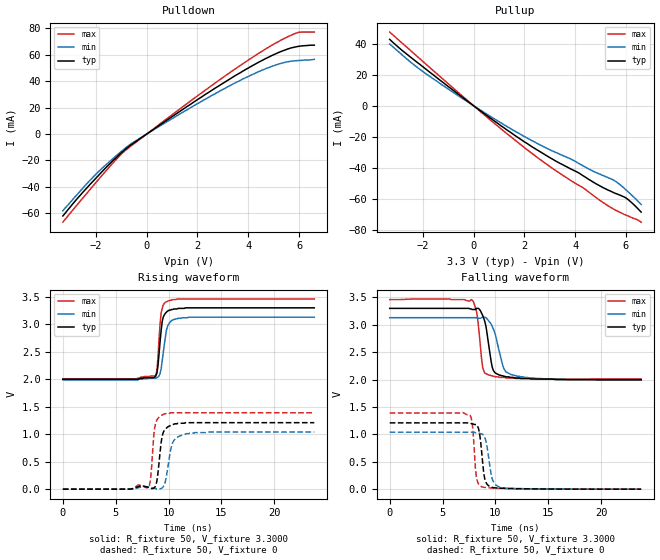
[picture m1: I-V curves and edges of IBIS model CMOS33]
|   IBIS Models For TG-5511CB (CMOS)
[IBIS Ver]   3.2
[File name]   tg5511cb_cmos.ibs
[File Rev]   1.0
[Date]   Feb 10, 2021
[Source]   From silicon level SPICE model at Seiko Epson.
[Notes]
[Disclaimer]
This information is for modeling purposes only, and is not guaranteed.
Property of SEIKO EPSON Corp.,
unauthorized reproduction and/or distribution is strictly prohibited.
[Copyright]   Copyright 2021, SEIKO EPSON Corp. All rights reserved.
[Component]   TG-5511CB (CMOS)
[Manufacturer] SEIKO EPSON Corp.
[Package]
| variable   typ   min   max
R_pkg   0.10   NA   NA
L_pkg   1.47n   NA   NA
C_pkg   0.81p   NA   NA
[Pin] signal_name   model_name   R_pin  L_pin  C_pin
  4   GND   GND   NA   NA   NA
  5   OUT   CMOS33   NA   NA   NA
  9   VCC   POWER   NA   NA   NA
| Models and submodels in the file (1): CMOS33 (Output)
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|   Model_type Output
[Model] CMOS33
Model_type  Output
Enable   Active-High
Polarity   Non-Inverting
Vmeas = 1.65
C_comp   2.5p   2.0p   3.0p
[Temperature Range]   25   85   -40
[Voltage Range]   3.3000   3.1350   3.4650
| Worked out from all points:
|   slope of the pulldown table from 0 to 0.495 V, typ, clamps not added: 75.5 ohm
|   slope of the pullup table from 0 to 0.495 V, typ, clamps not added: 82.4 ohm
|   falling waveform, R_fixture 50, V_fixture 3.3000: 20-80 % time 645ps typ, 914ps min, 467ps max; typ from 3.3 V to 2 V
|   falling waveform, R_fixture 50, V_fixture 0: 20-80 % time 408ps typ, 524ps min, 316ps max; typ from 1.21 V to 0 V
|   rising waveform, R_fixture 50, V_fixture 3.3000: 20-80 % time 385ps typ, 497ps min, 322ps max; typ from 2 V to 3.3 V
|   rising waveform, R_fixture 50, V_fixture 0: 20-80 % time 442ps typ, 594ps min, 343ps max; typ from 0 V to 1.21 V
[Pullup]
|   voltage   I(typ)   I(min)   I(max)
-3.3V     42.8mA     39.8mA     47.5mA
-2.2V     27.7mA     24.5mA     31.5mA
-1.3V     16.2mA     14.1mA     18.5mA
800mV     -9.64mA    -8.3mA     -11.1mA
2.5V      -28.5mA    -24.3mA    -33.3mA
3.2V      -35.4mA    -29.9mA    -41.5mA
3.9V      -41.4mA    -35mA      -49mA
4.4V      -46.1mA    -39.6mA    -54mA
4.8V      -50.2mA    -43mA      -59mA
5.5V      -56mA      -47.9mA    -66.6mA
6V        -59.5mA    -54.3mA    -70.6mA
6.6V      -68.7mA    -63.8mA    -75.2mA
[Pulldown]
|   voltage   I(typ)   I(min)   I(max)
-3.3V     -62mA      -58mA      -66.7mA
-2.7V     -48.1mA    -45mA      -52.7mA
-2V       -33.4mA    -30.4mA    -36.7mA
-1V       -14.2mA    -13.1mA    -15.2mA
-500mV    -6.65mA    -5.94mA    -7.33mA
1V        13.2mA     11.7mA     14.6mA
3.2V      40.8mA     35.9mA     45.5mA
4.2V      52.2mA     45.4mA     58.5mA
4.9V      59.2mA     51.1mA     66.9mA
5.4V      63.3mA     54.1mA     72.2mA
5.9V      66.1mA     55.6mA     76.5mA
6.6V      67.3mA     56.6mA     77.2mA
[Falling Waveform]
R_fixture = 50
V_fixture = 3.3000
V_fixture_min = 3.1350
V_fixture_max = 3.4650
0s        3.3V       3.13V      3.46V
7.8ns     3.28V      3.13V      3.45V
8.3ns     3.3V       3.12V      3.15V
8.8ns     3.17V      3.14V      2.22V
9.1ns     2.98V      3.13V      2.11V
9.4ns     2.59V      3.06V      2.08V
9.9ns     2.14V      2.88V      2.06V
10.8ns    2.06V      2.2V       2.04V
11.5ns    2.04V      2.09V      2.03V
23.8ns    2V         1.99V      2.01V
[Falling Waveform]
R_fixture = 50
V_fixture = 0
V_fixture_min = 0
V_fixture_max = 0
0s        1.21V      1.04V      1.39V
7.6ns     1.21V      1.04V      1.35V
7.8ns     1.19V      1.04V      1.22V
8.2ns     1.18V      1.03V      223mV
8.5ns     1.02V      1.02V      70.5mV
8.8ns     473mV      1V         38.4mV
9.1ns     127mV      882mV      29.5mV
9.7ns     32.7mV     189mV      20.5mV
10.4ns    18.8mV     39.6mV     14mV
23.8ns    67.4uV     246uV      17.2uV
[Rising Waveform]
R_fixture = 50
V_fixture = 3.3000
V_fixture_min = 3.1350
V_fixture_max = 3.4650
0s        2V         1.99V      2.01V
8.7ns     2.04V      2.02V      2.06V
8.9ns     2.11V      2.03V      2.15V
9.2ns     2.68V      2.1V       3.01V
9.3ns     2.88V      2.19V      3.2V
9.5ns     3.13V      2.48V      3.35V
9.8ns     3.22V      2.89V      3.41V
10ns      3.25V      3V         3.43V
11.9ns    3.3V       3.13V      3.46V
23.8ns    3.3V       3.13V      3.46V
[Rising Waveform]
R_fixture = 50
V_fixture = 0
V_fixture_min = 0
V_fixture_max = 0
0s        44.12uV    170uV      13.13uV
8.1ns     29.7mV     37.8mV     34.7mV
8.3ns     13.7mV     32mV       178mV
8.7ns     33.9mV     13.6mV     1.13V
8.9ns     146mV      5.26mV     1.26V
9.3ns     847mV      10.7mV     1.34V
9.6ns     1.07V      75.5mV     1.37V
10.4ns    1.18V      849mV      1.39V
11.4ns    1.2V       992mV      1.39V
23.8ns    1.21V      1.04V      1.39V
[Ramp]
| variable   typ   min   max
dV/dt_r   726.7m/0.444n   622.8m/0.591n   837.1m/0.346n
dV/dt_f   726.7m/0.407n   622.8m/0.523n   837.1m/0.319n
R_load = 50ohms
